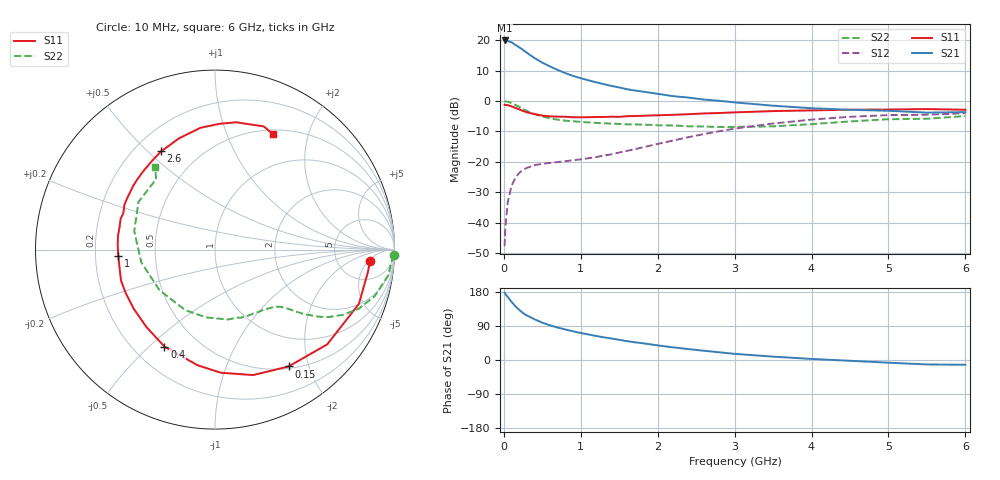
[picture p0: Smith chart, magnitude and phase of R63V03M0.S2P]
! SIEMENS Small Signal Semiconductors
! BFR193
! Si NPN RF Bipolar Junction Transistor in SOT23
! VCE = 3 V  IC = 3 mA
! Common Emitter S-Parameters:  May  1996
# GHz  S  MA  R  50
!  f  S11  S21  S12  S22
! GHz  MAG  ANG  MAG  ANG  MAG  ANG  MAG  ANG
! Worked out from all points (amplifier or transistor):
!   36 points, 10 MHz to 6 GHz, reference 50 ohm
!   highest |S21| = 19.9 dB at 10 MHz (marker M1)
!   |S21| within 3 dB of that: start of sweep to 243 MHz
!   unconditionally stable (mu >= 1): 1.045 GHz to 2.022 GHz
!   at 250 MHz: K = 0.31, MSG = 19.7 dB, |S12| = -22.6 dB
!   at 1.4 GHz: K = 1.09, MAG = 9.4 dB, |S12| = -17.5 dB
!   at 6 GHz: K = 0.98, MSG = 0.2 dB, |S12| = -4.0 dB
!   S11 on the Smith chart (normalised r, x): 10 MHz: 11, -6; 150 MHz: 0.53, -1.69; 400 MHz: 0.32, -0.56; 1 GHz: 0.30, -0.03; 2.6 GHz: 0.31, +0.55; 6 GHz: 0.56, +1.48
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0.01  0.8661 -4.2  9.921 177.5  0.0041 88.3  0.9953 -1.7
0.02  0.8613 -8.3  9.84 174.4  0.0086 83.6  0.9868 -3.5
0.05  0.8569 -20.7  9.68 166.5  0.0214 79.1  0.9759 -8.5
0.1  0.8183 -40.2  9.267 153.6  0.0403 69.6  0.9265 -16.3
0.15  0.7694 -57.8  8.385 141.9  0.0547 61.1  0.8646 -22.5
0.2  0.7306 -73.1  7.667 132.3  0.0659 54.8  0.8 -27.0
0.25  0.6867 -87.3  6.924 123.9  0.0738 49.8  0.7361 -30.7
0.3  0.6518 -98.5  6.204 117.4  0.0796 46.5  0.6839 -33.1
0.4  0.6096 -117.5  5.09 107.3  0.0882 41.8  0.6105 -36.0
0.5  0.5761 -131.6  4.28 98.5  0.0929 39.6  0.5569 -37.8
0.6  0.56 -143.9  3.704 91.5  0.0961 39.6  0.5185 -39.2
0.7  0.5533 -154.1  3.248 85.6  0.0992 40.0  0.4933 -40.6
0.8  0.5513 -161.7  2.874 80.5  0.1026 40.9  0.4756 -42.0
1  0.5401 -176.3  2.373 71.3  0.1097 44.6  0.4541 -45.1
1.1  0.5426 177.6  2.191 67.4  0.1147 46.9  0.4446 -47.4
1.6  0.563 153.7  1.566 49.8  0.1515 56.9  0.4146 -59.6
2.2  0.5934 131.6  1.203 33.4  0.2243 60.2  0.3963 -79.4
2.6  0.6246 118.7  1.058 24.5  0.2859 57.5  0.3809 -96.3
3.5  0.6836 96.8  0.838 8.9  0.4271 43.6  0.3833 -143.8
4.5  0.7192 80.5  0.718 -2.1  0.5509 24.5  0.4615 167.1
5.5  0.7382 68.4  0.645 -11.7  0.5951 6.2  0.5114 129.9
6  0.719 63.2  0.657 -12.6  0.631 1.0  0.5664 126.0
